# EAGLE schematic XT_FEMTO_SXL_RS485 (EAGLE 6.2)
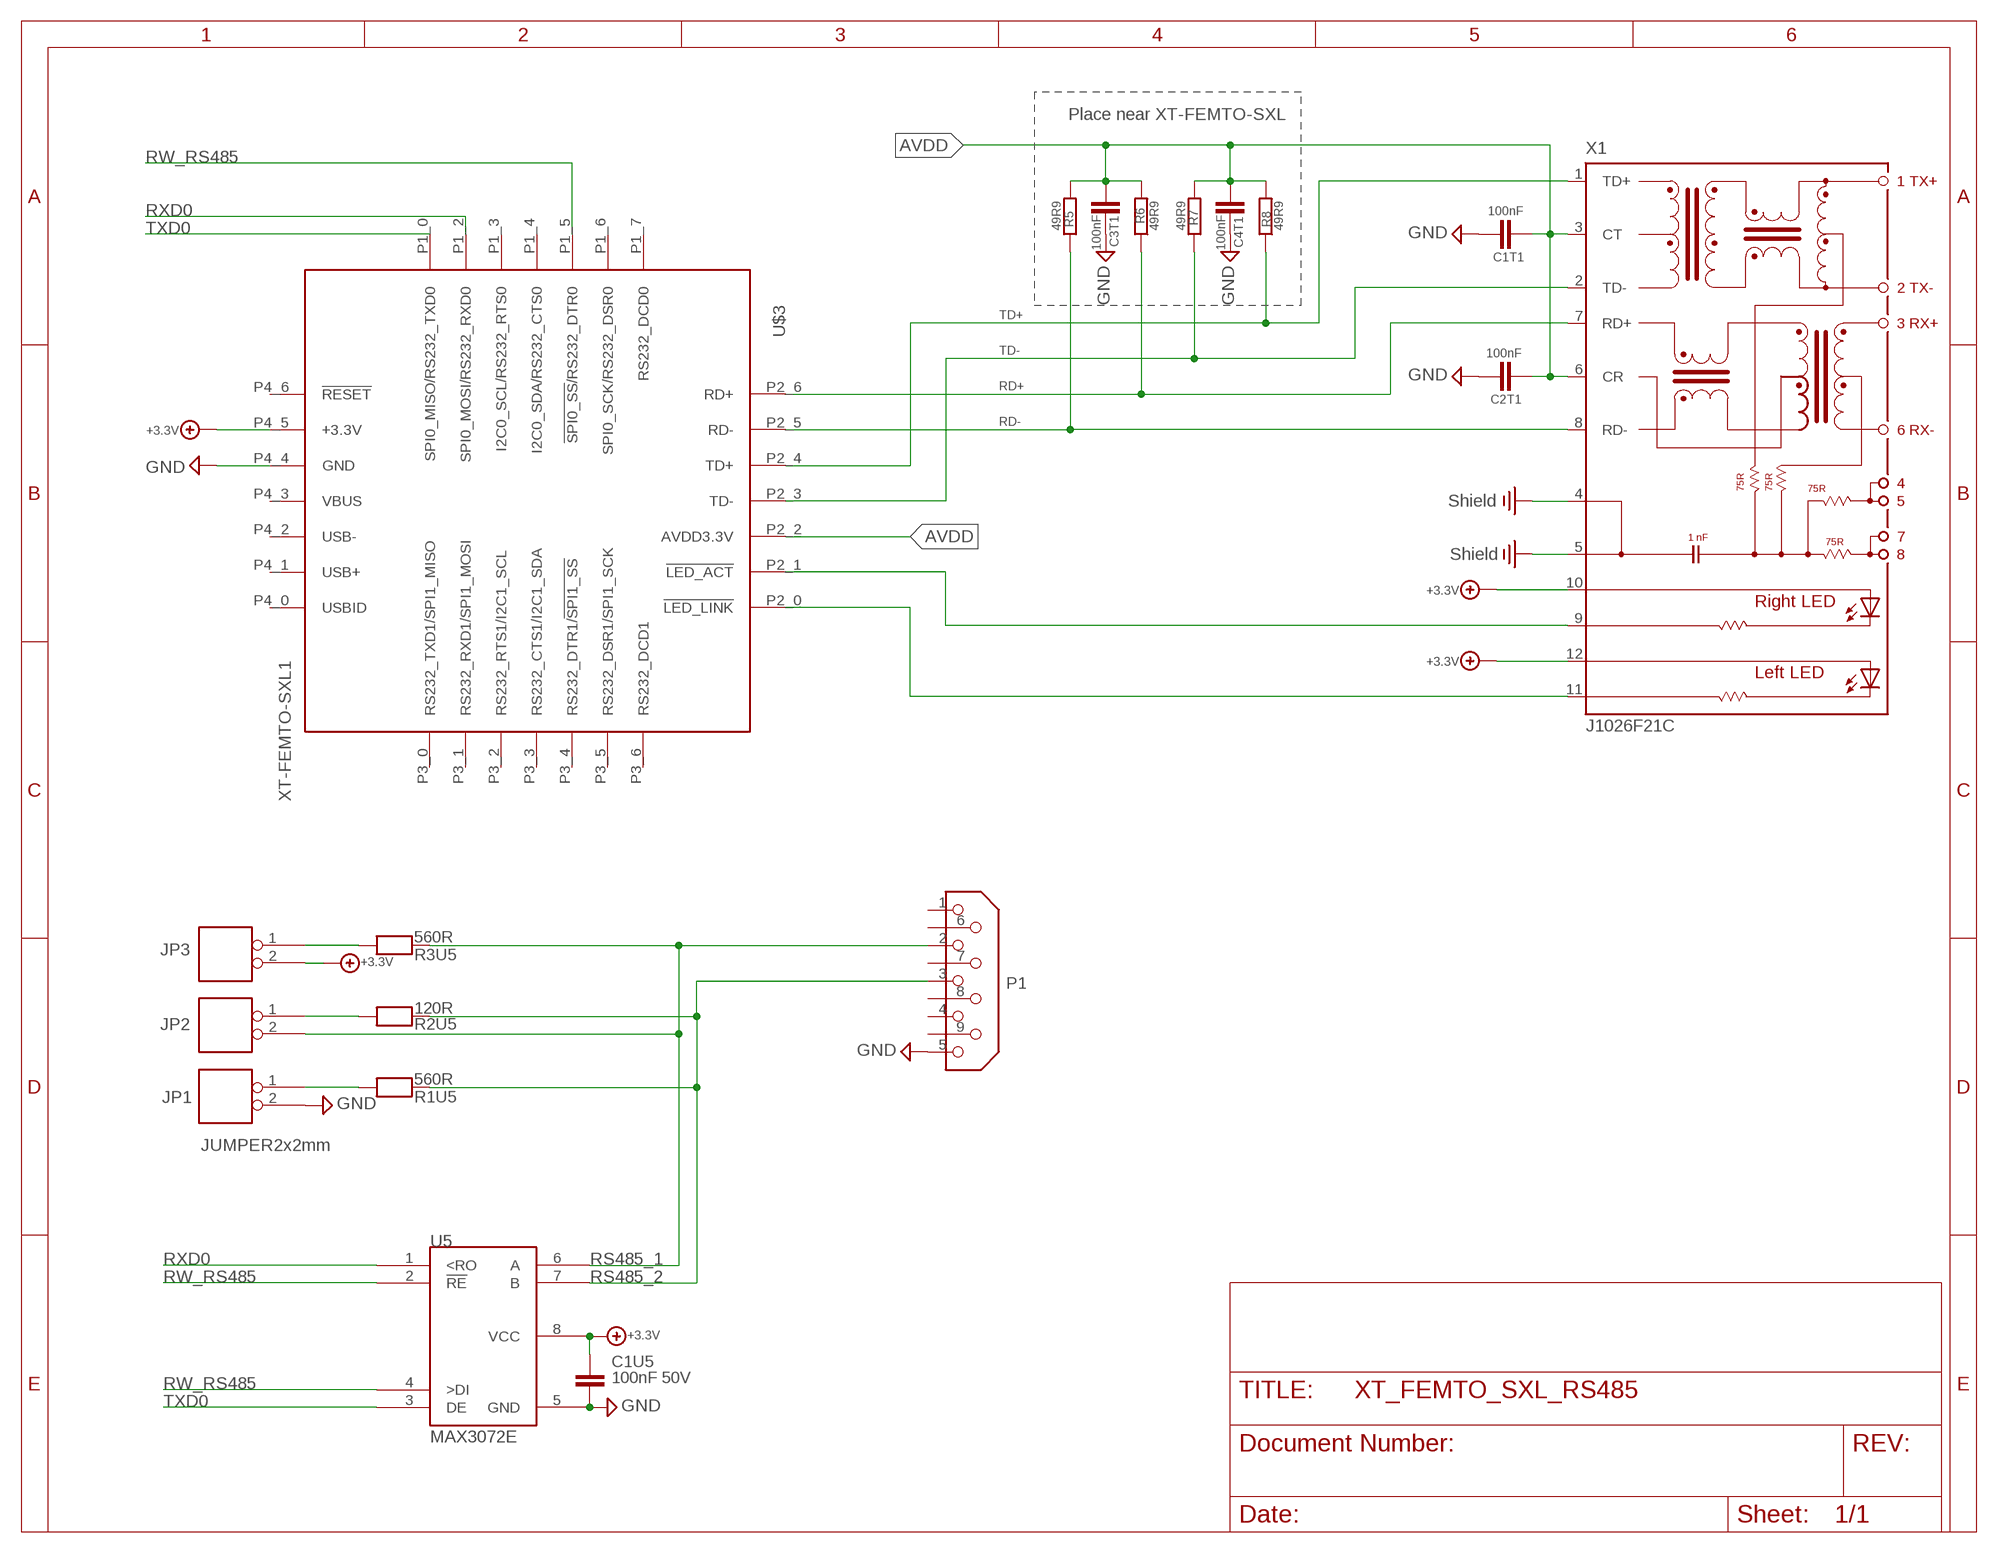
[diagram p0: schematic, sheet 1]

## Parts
C1T1  100nF  CHIP-C-VTS0402  [R0402_VTS]
C1U5  100nF 50V  CHIP-C-0603  [SMD-0603]
C2T1  100nF  CHIP-C-VTS0402  [R0402_VTS]
C3T1  100nF  CHIP-C-VTS0402  [R0402_VTS]
C4T1  100nF  CHIP-C-VTS0402  [R0402_VTS]
JP1  JUMPER2x2mm  JP2  [ROLF_SQW1X2]
JP2  JUMPER2x2mm  JP2  [ROLF_SQW1X2]
JP3  JUMPER2x2mm  JP2  [ROLF_SQW1X2]
P1  DB9  [MSUB9-5]
R1U5  560R  CHIP-R-0603  [SMD-0603@1]
R2U5  120R  CHIP-R-0603  [SMD-0603@1]
R3U5  560R  CHIP-R-0603  [SMD-0603@1]
R5  49R9  R-EU_R0603  [R0603]
R6  49R9  R-EU_R0603  [R0603]
R7  49R9  R-EU_R0603  [R0603]
R8  49R9  R-EU_R0603  [R0603]
U5  MAX3072E  MAX3072E_SO8  [SO-8]
U$3  XT-FEMTO-SXL1  [XT-FEMTO-SXL-PIN]
X1  J1026F21C  [J1]

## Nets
+3.3V: C1U5.2 JP3.2 U5.8(VCC) U$3.P4_5(+3.3V) X1.10(A-R) X1.12(A-L)
AVDD: C1T1.1 C2T1.2 C3T1.1 C4T1.2 R5.2 R6.2 R7.2 R8.2 U$3.P2_2(AVDD3.3V) X1.3(CT) X1.6(CR)
GND: C1T1.2 C1U5.1 C2T1.1 C3T1.2 C4T1.1 JP1.2 P1.5 U5.5(GND) U$3.P4_4(GND)
N14469550: JP2.1 R2U5.2
N15158340: JP1.1 R1U5.2
N15158360: JP3.1 R3U5.2
N$3: U$3.P2_1(!LED_ACT) X1.9(C-R)
N$5: U$3.P2_0(!LED_LINK) X1.11(C-L)
PE: X1.4 X1.5 ; supply symbol labelled Shield
RD+: R6.1 U$3.P2_6(RD+) X1.7(RD+)
RD-: R5.1 U$3.P2_5(RD-) X1.8(RD-)
RS485_1: JP2.2 P1.2 R3U5.1 U5.6(A)
RS485_2: P1.3 R1U5.1 R2U5.1 U5.7(B)
RW_RS485: U5.2(!RE) U5.4(>DI) U$3.P1_5(!SPI0_SS!/RS232_DTR0)
RXD0: U5.1(<RO) U$3.P1_2(SPI0_MOSI/RS232_RXD0)
TD+: R8.1 U$3.P2_4(TD+) X1.1(TD+)
TD-: R7.1 U$3.P2_3(TD-) X1.2(TD-)
TXD0: U5.3(DE) U$3.P1_0(SPI0_MISO/RS232_TXD0)
Unconnected: P1.1 P1.4 P1.6 P1.7 P1.8 P1.9 U$3.P1_3(I2C0_SCL/RS232_RTS0) U$3.P1_4(I2C0_SDA/RS232_CTS0) U$3.P1_6(SPI0_SCK/RS232_DSR0) U$3.P1_7(RS232_DCD0) U$3.P3_0(RS232_TXD1/SPI1_MISO) U$3.P3_1(RS232_RXD1/SPI1_MOSI) U$3.P3_2(RS232_RTS1/I2C1_SCL) U$3.P3_3(RS232_CTS1/I2C1_SDA) U$3.P3_4(RS232_DTR1/!SPI1_SS!) U$3.P3_5(RS232_DSR1/SPI1_SCK) U$3.P3_6(RS232_DCD1) U$3.P4_0(USBID) U$3.P4_1(USB+) U$3.P4_2(USB-) U$3.P4_3(VBUS) U$3.P4_6(!RESET)

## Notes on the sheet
- Place near XT-FEMTO-SXL

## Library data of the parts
C1T1 C1U5 C2T1 C3T1 C4T1 = mea-lib:CHIP-C-?: Chip capacitance
JP1-JP3 = XTMACRO_AS:JP2
P1 = XTMACRO:DB9
R1U5 R2U5 R3U5 = mea-lib:CHIP-R-?: Chip resistors
R5-R8 = rcl:R-EU_: RESISTOR, European symbol
U5 = XTMACRO_AS:MAX3072E_SO8
U$3 = ak-devices:XT-FEMTO-SXL: AK-NORD XT-FEMTO-SXL
X1 = con-pulse:J1026F: PULSEJACK (TM) 1x1 Tab-UP RJ45 10/100 Base-TX RJ45 1x1 Tab-UP with LEDs 8-pin (J1 series) and 6-pin (JP series) integrated magnetics connector, designed to support applications, such as ADSL modems, LAN-on-Motherboard, and Hub and Switches. Source: www.pulseeng.com .. PulseJack-J402.pdf; OC_FARNELL: unknown; OC_NEWARK: unknown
